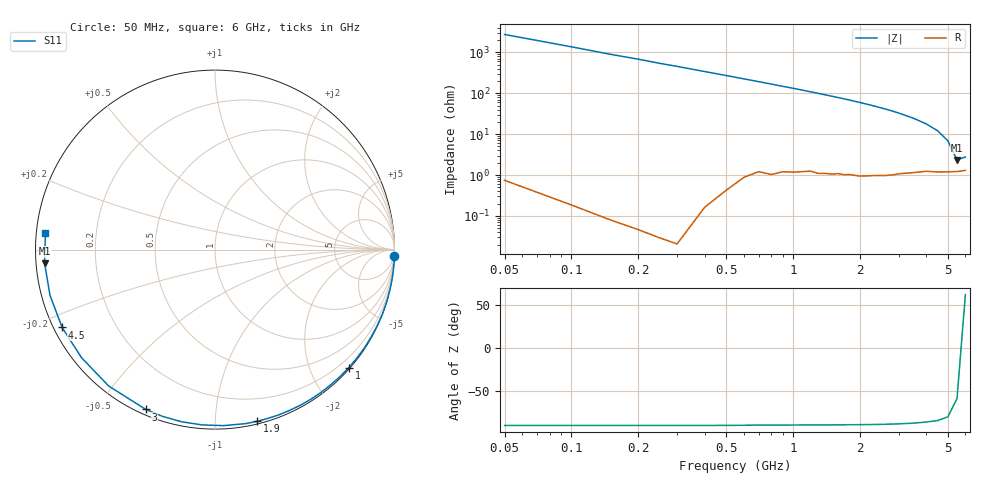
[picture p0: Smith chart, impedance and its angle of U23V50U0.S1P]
! SIEMENS Discrete & RF Semiconductors
! BBY52-02W
! Si Tuning Diode in SCD-80
! VR = 3.5 V
! S-Parameters:  September  1997
# GHz  S  MA  R  50
!  f  S11
! GHz  MAG  ANG
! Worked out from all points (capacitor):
!   34 points, 50 MHz to 6 GHz, reference 50 ohm
!   read as one part to ground: C = 1.17 pF near 50 MHz
!   lowest |Z| = 2.35 ohm at 5.5 GHz (marker M1)
!   series resonance near 5.725 GHz, so ESL is about 660 pH
!   S11 on the Smith chart (normalised r, x): 50 MHz: 0, -55; 1 GHz: 0.02, -2.65; 1.9 GHz: 0.02, -1.27; 3 GHz: 0.02, -0.66; 4.5 GHz: 0.02, -0.24; 6 GHz: 0.03, +0.05
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0.05  1 -2.1
0.2  1 -8.4
0.3  1 -12.6
0.4  0.9999 -16.8
0.5  0.9994 -20.9
0.6  0.9983 -25.1
0.8  0.9966 -33.3
0.9  0.995 -37.5
1  0.9941 -41.4
1.1  0.9928 -45.5
1.3  0.9912 -53.4
1.5  0.9891 -61.3
1.6  0.9875 -65.1
1.7  0.987 -68.8
1.8  0.9856 -72.7
1.9  0.9851 -76.3
2  0.9845 -80.0
2.2  0.9819 -87.2
2.4  0.9793 -94.1
2.6  0.9771 -100.8
2.8  0.9742 -107.3
3  0.9704 -113.4
3.5  0.9636 -127.9
4  0.9569 -141.0
4.5  0.9559 -153.0
5  0.9539 -164.5
5.5  0.9525 -175.4
6  0.9494 174.4
